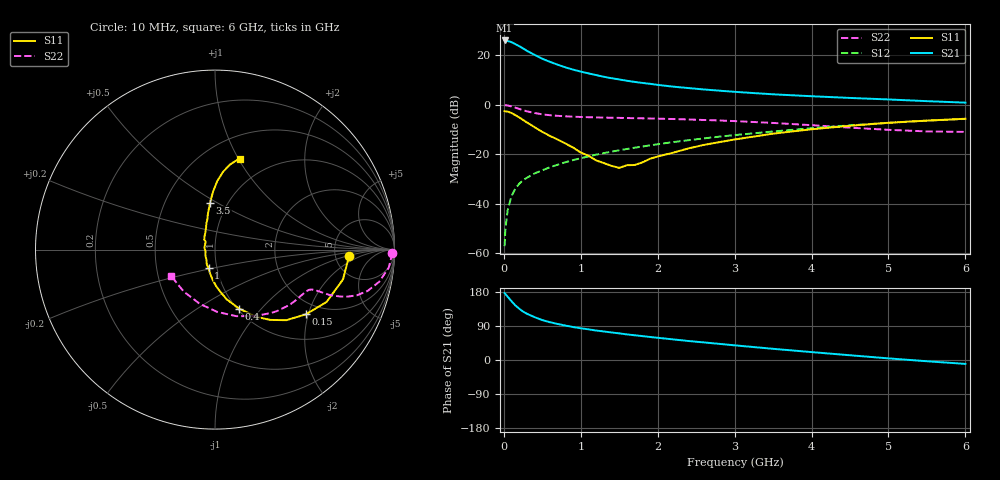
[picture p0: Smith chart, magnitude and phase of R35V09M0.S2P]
! SIEMENS Small Signal Semiconductors
! BFR181
! Si NPN RF Bipolar Junction Transistor in SOT23
! VCE = 5 V  IC = 9 mA
! Common Emitter S-Parameters:  May  1996
# GHz  S  MA  R  50
!  f  S11  S21  S12  S22
! GHz  MAG  ANG  MAG  ANG  MAG  ANG  MAG  ANG
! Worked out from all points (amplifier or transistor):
!   36 points, 10 MHz to 6 GHz, reference 50 ohm
!   highest |S21| = 26.1 dB at 10 MHz (marker M1)
!   |S21| within 3 dB of that: start of sweep to 237.7 MHz
!   unconditionally stable (mu >= 1): 870.8 MHz to 2.73 GHz
!   at 250 MHz: K = 0.57, MSG = 26.6 dB, |S12| = -30.4 dB
!   at 1.4 GHz: K = 1.05, MAG = 13.4 dB, |S12| = -18.9 dB
!   at 6 GHz: K = 0.86, MSG = 3.3 dB, |S12| = -5.6 dB
!   S11 on the Smith chart (normalised r, x): 10 MHz: 6.74, -1.03; 150 MHz: 1.64, -1.93; 400 MHz: 1.02, -0.77; 1 GHz: 0.91, -0.19; 3.5 GHz: 0.83, +0.47; 6 GHz: 0.72, +1.01
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0.01  0.7468 -2.6  20.07 176.8  0.0014 97.2  0.9863 -1.1
0.02  0.7422 -5.0  19.69 174.2  0.0031 84.4  0.9838 -2.4
0.05  0.7323 -13.1  19.59 166.8  0.0075 83.6  0.9733 -5.9
0.1  0.687 -25.1  18.57 155.1  0.0145 77.5  0.9322 -11.1
0.15  0.6212 -35.5  16.89 144.0  0.0203 73.3  0.8803 -15.2
0.2  0.559 -44.7  15.4 135.4  0.0256 71.6  0.8297 -17.9
0.25  0.4986 -51.8  13.84 127.8  0.0301 69.2  0.7816 -19.6
0.3  0.4424 -58.1  12.41 122.0  0.0338 68.8  0.7427 -20.6
0.4  0.3551 -67.8  10.25 113.1  0.0413 67.6  0.6868 -21.6
0.5  0.2853 -76.7  8.575 105.3  0.0477 67.9  0.6463 -21.8
0.6  0.2362 -82.9  7.411 99.7  0.0552 68.5  0.6191 -21.9
0.7  0.1998 -88.9  6.494 95.0  0.0619 69.0  0.6018 -22.1
0.8  0.1665 -94.9  5.751 90.8  0.0695 68.9  0.5886 -22.3
1  0.1091 -109.2  4.713 83.7  0.0837 69.2  0.5708 -23.1
1.1  0.0942 -119.0  4.341 80.9  0.0911 69.3  0.5647 -23.8
1.3  0.0668 -140.2  3.71 75.3  0.1063 69.1  0.5546 -25.3
1.6  0.0604 169.0  3.075 67.5  0.129 67.9  0.5431 -28.3
2.2  0.1083 120.0  2.341 54.4  0.1772 64.8  0.519 -35.8
3.5  0.2629 96.0  1.638 29.5  0.2908 54.5  0.4326 -58.9
4.5  0.3793 88.3  1.384 12.5  0.3867 43.7  0.3475 -87.9
5.5  0.4824 79.9  1.192 -3.3  0.4802 31.1  0.2915 -126.7
6  0.5255 74.9  1.112 -10.3  0.5222 24.2  0.285 -148.6
